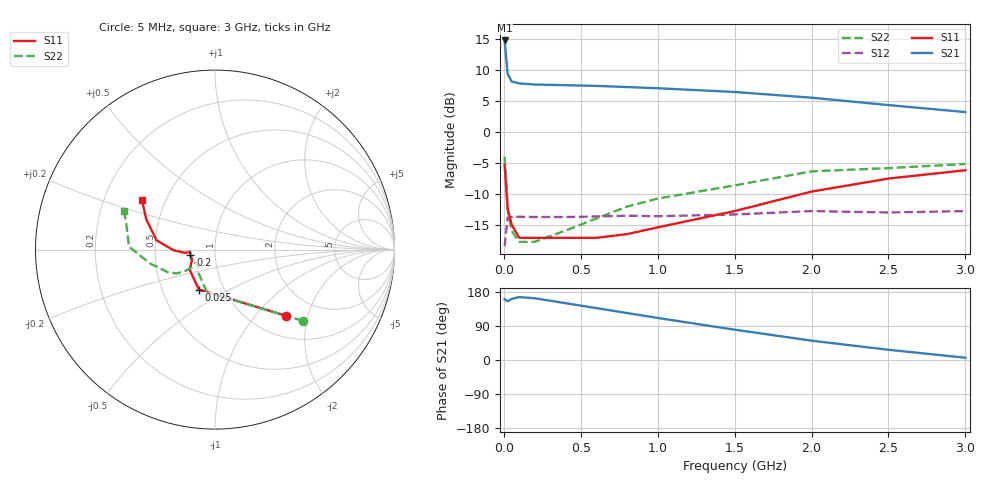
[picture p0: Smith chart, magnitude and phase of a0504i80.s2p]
!  MSA-0504 S PARAMETERS
!  Id=80 mA  LAST UPDATED 07-22-92
# ghz s ma r 50
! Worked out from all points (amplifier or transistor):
!   13 points, 5 MHz to 3 GHz, reference 50 ohm
!   highest |S21| = 14.7 dB at 5 MHz (marker M1)
!   |S21| within 3 dB of that: start of sweep to 16.14 MHz
!   unconditionally stable (mu >= 1): 26.29 MHz to 1.793 GHz
!   at 50 MHz: K = 1.15, MAG = 8.5 dB, |S12| = -13.7 dB
!   at 600 MHz: K = 1.21, MAG = 7.7 dB, |S12| = -13.6 dB
!   at 3 GHz: K = 0.80, MSG = 8.0 dB, |S12| = -12.8 dB
!   S11 on the Smith chart (normalised r, x): 5 MHz: 1.41, -1.47; 25 MHz: 0.76, -0.36; 200 MHz: 0.76, -0.05; 3 GHz: 0.37, +0.27
0.005  0.54 -43.0  5.43 160.0  0.12 37.0  0.63 -39.0
0.025  0.24 -112.0  2.92 155.0  0.204 12.0  0.24 -101.0
0.05  0.18 -142.0  2.54 161.0  0.206 3.0  0.16 -125.0
0.1  0.14 -156.0  2.45 166.0  0.207 3.0  0.13 -137.0
0.2  0.14 -168.0  2.4 163.0  0.206 1.0  0.13 -146.0
0.4  0.14 -174.0  2.37 150.0  0.206 1.0  0.16 -143.0
0.6  0.14 -175.0  2.34 137.0  0.208 -1.0  0.2 -144.0
0.8  0.15 -174.0  2.29 124.0  0.211 -1.0  0.25 -148.0
1  0.17 -174.0  2.24 111.0  0.209 -3.0  0.29 -154.0
1.5  0.23 -179.0  2.09 80.0  0.216 -4.0  0.37 -168.0
2  0.33 171.0  1.88 51.0  0.23 -10.0  0.48 178.0
2.5  0.42 156.0  1.64 27.0  0.224 -12.0  0.51 165.0
3  0.49 146.0  1.44 6.0  0.23 -11.0  0.55 157.0
